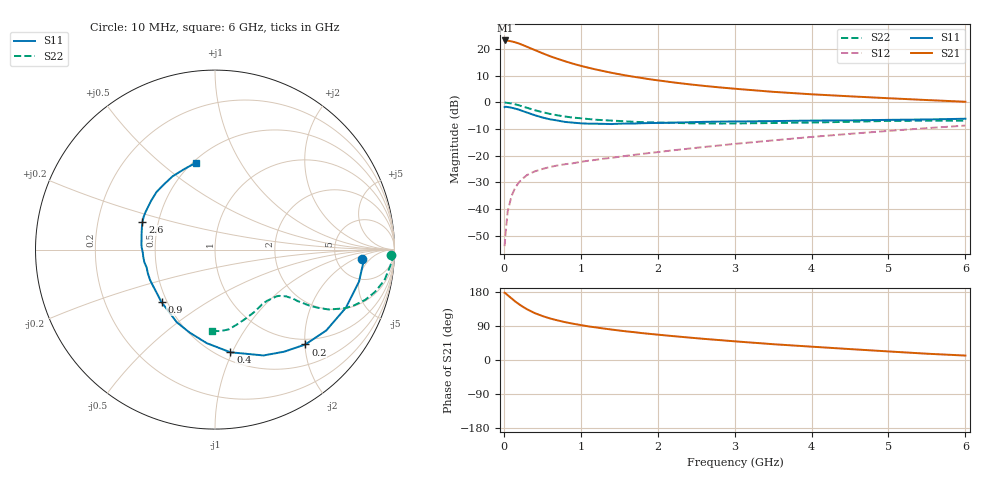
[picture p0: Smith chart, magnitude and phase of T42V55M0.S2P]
! Infineon Technologies  Discrete & RF Semiconductors
! BFR182T
! Si NPN RF Bipolar Junction Transistor in SC75
! VCE = 2.5 V  IC = 5 mA
! Common Emitter S-Parameters:  October  1999
# GHz  S  MA  R  50
!  f  S11  S21  S12  S22
! GHz  MAG  ANG  MAG  ANG  MAG  ANG  MAG  ANG
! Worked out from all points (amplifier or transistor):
!   36 points, 10 MHz to 6 GHz, reference 50 ohm
!   highest |S21| = 23.3 dB at 20 MHz (marker M1)
!   |S21| within 3 dB of that: start of sweep to 352.7 MHz
!   unconditionally stable (mu >= 1): 1.367 GHz to 4.01 GHz
!   at 250 MHz: K = 0.28, MSG = 25.0 dB, |S12| = -28.5 dB
!   at 1.4 GHz: K = 1.01, MAG = 15.3 dB, |S12| = -20.8 dB
!   at 6 GHz: K = 0.84, MSG = 4.5 dB, |S12| = -8.7 dB
!   lowest NFmin = 1.20 dB at 450 MHz
!   S11 on the Smith chart (normalised r, x): 10 MHz: 9.12, -2.84; 200 MHz: 0.89, -2.01; 400 MHz: 0.57, -0.98; 900 MHz: 0.47, -0.33; 2.6 GHz: 0.41, +0.16; 6 GHz: 0.52, +0.66
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0.01  0.8183 -3.6  14.54 177.4  0.002 87.2  0.9834 -1.8
0.02  0.8324 -3.6  14.64 176.6  0.0032 94.9  0.9952 -2.2
0.05  0.8221 -12.5  14.5 171.0  0.009 86.1  0.981 -5.3
0.1  0.798 -23.9  14.07 162.6  0.0175 79.4  0.9591 -10.3
0.15  0.7663 -36.0  13.49 154.1  0.0255 72.6  0.9222 -14.8
0.2  0.7298 -46.4  12.77 146.8  0.0321 69.4  0.8828 -18.5
0.25  0.687 -55.9  11.95 140.1  0.0376 64.4  0.8372 -21.7
0.3  0.6486 -65.4  11.15 134.1  0.0433 60.8  0.7964 -24.2
0.4  0.5784 -81.5  9.704 123.9  0.0507 55.8  0.7186 -27.7
0.5  0.5231 -95.1  8.449 116.2  0.0563 53.6  0.6583 -29.5
0.6  0.4832 -107.1  7.413 109.6  0.0615 52.3  0.6113 -30.7
0.7  0.4575 -117.7  6.602 104.4  0.0657 51.8  0.5734 -31.3
0.8  0.4308 -126.8  5.929 99.7  0.0694 51.5  0.5443 -31.9
0.9  0.4184 -135.4  5.349 95.8  0.0722 52.1  0.5202 -32.1
1.1  0.4002 -149.4  4.499 88.7  0.0806 53.5  0.489 -32.9
1.6  0.4019 -174.6  3.197 75.4  0.1 56.8  0.4404 -35.8
2.2  0.4184 167.8  2.389 63.0  0.1265 59.8  0.4145 -41.8
2.6  0.4327 159.0  2.054 55.8  0.146 61.1  0.404 -46.6
3.5  0.4477 142.9  1.587 41.7  0.1942 61.4  0.4115 -58.6
4.5  0.4613 128.2  1.306 28.8  0.2579 58.9  0.4339 -73.1
5.5  0.48 111.0  1.112 16.6  0.3301 54.2  0.4551 -86.4
6  0.4955 102.4  1.033 11.7  0.3683 50.8  0.4532 -92.1
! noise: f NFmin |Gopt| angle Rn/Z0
0.45  1.2  0.27  37  0.3
0.9  1.3  0.25  75  0.23
1.8  1.9  0.21  145  0.2
